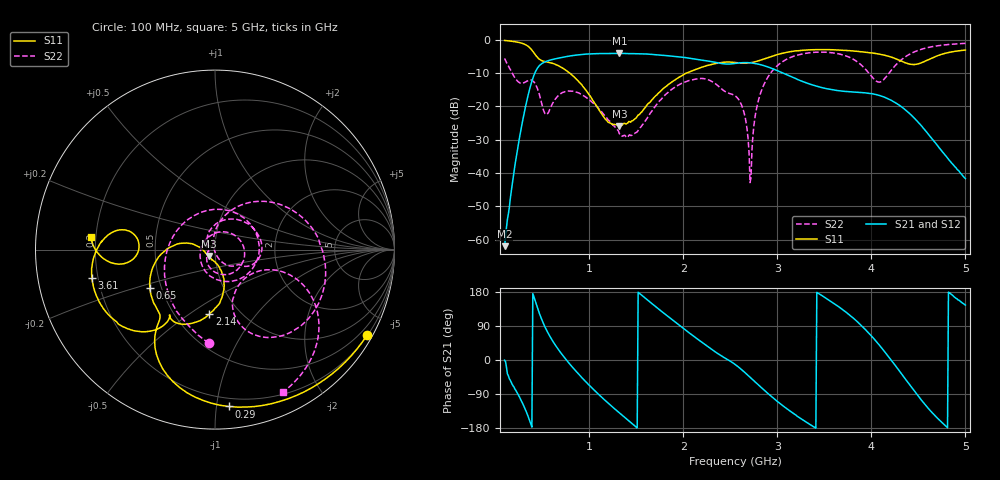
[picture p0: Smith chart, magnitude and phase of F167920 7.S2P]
!  2-Port S-parameters saved by WinCal
! VAR MeasName=S-Parameters (CALIBRATED_DATA) read from VNA (N5242A)
! VAR MeasDate=2016-11-22 9:53:50
! VAR NAME=F167920 7
! VAR FILENAME=F167920 7.S2P
! VAR DATE=2016-11-22 9:53:50
! VAR PHYS_PORTS=1,2
# Hz S DB R 50
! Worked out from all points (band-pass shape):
!   491 points, 100 MHz to 5 GHz, reference 50 ohm
!   highest |S21| = -4.12 dB at 1.32 GHz (marker M1); lowest = -61.9 dB at 100 MHz (marker M2)
!   |S21| within 3 dB of the highest: 499.6 MHz to 2.398 GHz (1.898 GHz wide, 131 % of centre); 2.556 GHz to 2.756 GHz (200 MHz wide, 7.53 % of centre)
!   lowest |S11| = -26.0 dB at 1.32 GHz (marker M3), VSWR 1.11, Z = 46.5 - j3.27 ohm
!   |S11| at or under -10 dB: 791.9 MHz to 2.036 GHz (1.244 GHz wide, 88 % of centre)
!   |S22| runs from -42.8 to -1.1 dB; largest |S21 - S12| = 0.0018
!   S11 on the Smith chart (normalised r, x): 100 MHz: 0.22, -3.82; 290 MHz: 0.14, -1.08; 650 MHz: 0.43, -0.22; 2.14 GHz: 0.73, -0.60; 3.61 GHz: 0.18, -0.11; 5 GHz: 0.18, +0.05
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1e8  -0.25 -29.3  -61.90 -0.5  -62.17 1.3  -5.63 -93.8
1.9e8  -0.54 -55.1  -41.53 -68.1  -41.56 -67.4  -10.55 -161.4
2.9e8  -1.14 -85.1  -24.56 -113.7  -24.53 -113.7  -13.04 100.7
3.7e8  -2.50 -110.7  -14.42 -162.5  -14.41 -162.5  -12.13 14.6
4.4e8  -5.01 -126.0  -8.97 144.7  -8.96 144.7  -14.09 -64.3
5.4e8  -6.63 -133.0  -6.54 81.8  -6.54 81.8  -22.45 150.6
6.5e8  -7.53 -149.8  -5.68 35.4  -5.68 35.4  -17.42 37.0
9.2e8  -13.49 171.4  -4.43 -46.0  -4.43 -46.0  -16.48 -68.6
1.32e9  -26.03 -135.3  -4.12 -139.4  -4.11 -139.5  -28.15 -164.7
1.74e9  -15.92 -73.1  -4.58 134.2  -4.58 134.1  -18.60 101.2
2.14e9  -8.86 -94.9  -5.91 57.2  -5.90 57.2  -11.79 15.1
2.55e9  -6.86 -123.4  -7.13 -11.5  -7.12 -11.6  -16.82 -38.5
2.65e9  -7.08 -124.8  -6.89 -31.9  -6.87 -31.9  -22.30 -61.5
2.71e9  -6.95 -124.1  -6.95 -45.4  -6.93 -45.5  -42.85 -106.3
2.78e9  -6.51 -123.5  -7.24 -61.5  -7.22 -61.5  -20.50 91.0
2.89e9  -5.48 -125.1  -8.10 -86.2  -8.06 -86.3  -11.68 63.9
3.37e9  -3.03 -153.6  -13.55 -173.7  -13.52 -174.0  -3.85 -18.2
3.61e9  -3.05 -167.1  -15.13 148.0  -15.14 147.7  -4.04 -46.4
3.95e9  -3.83 177.4  -16.01 76.8  -16.00 76.5  -9.25 -73.2
4.19e9  -5.04 169.1  -17.89 6.5  -17.90 6.1  -9.95 -20.7
4.51e9  -7.16 -176.1  -25.11 -99.0  -25.15 -99.3  -3.10 -34.4
5e9  -3.14 174.2  -41.60 144.9  -41.61 144.1  -1.11 -64.5
